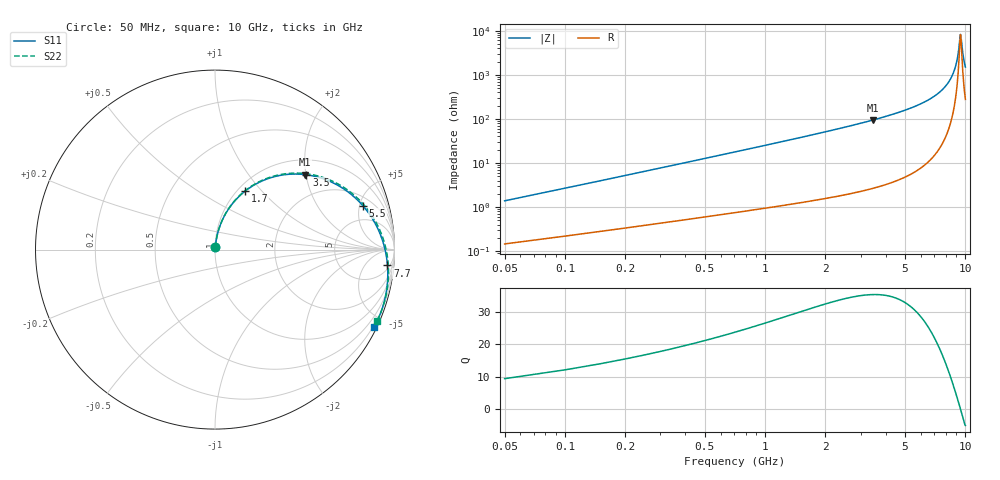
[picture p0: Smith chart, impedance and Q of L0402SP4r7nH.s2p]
!	AVX Thin Film Operation
!	Date:		5 January 2004
!	Description: 	Accu-L®  L0402 Series Thin Film RF Inductors
!	Part Number:	L04024R7AHLTR
!	50 MHz-20GHz Serial Measurements
#	mhz	S	db	R	50
!	S11	S11	S21	S21	S12	S12	S22	S22
!	dB	Phase	dB	Phase	dB	Phase	dB	Phase
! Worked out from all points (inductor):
!   200 points, 50 MHz to 10 GHz, reference 50 ohm
!   read as one part in series: L = 4.19 nH near 100 MHz
!   highest Q = 35.3 at 3.45 GHz (marker M1), where L = 4.34 nH
!   self-resonance near 9.45 GHz
!   S11 on the Smith chart (normalised r, x): 50 MHz: 1.00, +0.03; 1.7 GHz: 1.08, +0.82; 3.5 GHz: 1.37, +2.01; 5.5 GHz: 2.87, +5.37; 7.7 GHz: 7, -19; 10 GHz: 0.13, -4.32
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50  -37.74 82.7  -0.01 -0.8  -0.01 -0.8  -37.74 82.7
100  -32.07 83.3  -0.02 -1.6  -0.02 -1.6  -32.07 83.3
200  -26.33 82.8  -0.04 -3.2  -0.04 -3.2  -26.33 82.9
450  -19.57 79.9  -0.10 -7.0  -0.10 -7.0  -19.57 80.0
950  -13.38 73.1  -0.28 -14.4  -0.28 -14.4  -13.38 73.3
1700  -8.72 62.7  -0.74 -25.1  -0.74 -25.1  -8.72 63.1
1750  -8.50 62.0  -0.78 -25.8  -0.78 -25.8  -8.50 62.4
3400  -3.81 40.5  -2.56 -47.4  -2.56 -47.4  -3.81 41.2
3450  -3.72 39.9  -2.63 -48.0  -2.63 -48.0  -3.72 40.6
3500  -3.63 39.3  -2.70 -48.6  -2.70 -48.6  -3.63 40.0
5050  -1.68 21.4  -5.34 -66.2  -5.34 -66.2  -1.68 22.5
5500  -1.32 16.6  -6.32 -70.9  -6.32 -70.9  -1.32 17.8
6700  -0.64 4.3  -9.59 -82.4  -9.59 -82.4  -0.64 5.8
7700  -0.31 -5.3  -13.62 -90.8  -13.62 -90.8  -0.31 -3.5
8350  -0.18 -11.3  -17.70 -94.9  -17.70 -94.9  -0.18 -9.4
8700  -0.14 -14.5  -21.01 -95.7  -21.01 -95.7  -0.14 -12.5
9000  -0.12 -17.2  -25.30 -93.5  -25.30 -93.5  -0.12 -15.1
9200  -0.11 -19.0  -29.90 -86.3  -29.90 -86.3  -0.11 -16.8
9450  -0.10 -21.2  -38.64 -24.4  -38.64 -24.4  -0.10 -19.0
9500  -0.10 -21.6  -37.98 2.2  -37.98 2.2  -0.10 -19.4
9750  -0.11 -23.8  -29.02 48.3  -29.02 48.3  -0.11 -21.6
10000  -0.12 -26.0  -24.04 54.7  -24.04 54.7  -0.12 -23.7
